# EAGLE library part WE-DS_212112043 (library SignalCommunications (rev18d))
WE-DS D-SUB-Filter Connectors Bent 90° Characteristics Standard type filtered with 1000 pF High attenuation of more than 40 dB @ 180 MHz Choice of earthing metal sheet or high speed earthing clip Rated voltage: 100 VDC Rated current @ 20 ºC: 5 A Withstand voltage: 250 VRMS Insulation resistance: min. 1000 MΩ Operating temperature: –55 ºC to +125 ºC Applications Filtering of interfaces External connection to -printer -sensor -display Details see: http://katalog.we-online.de/en/pbs/Filter_abgewinkelt Created on 2015-05-04 2015 (C) Wurth Elektronik
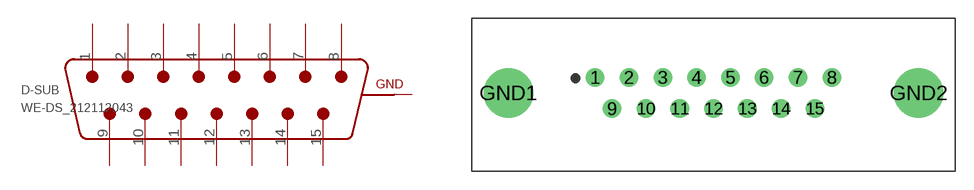
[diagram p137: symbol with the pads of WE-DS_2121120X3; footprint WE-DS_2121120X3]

Designator prefix D-SUB

## WE-DS_212112043 (WE-NUMBER: 212112043/15pins_male)  [WE-DS_2121120X3]
1  1  pas
2  2  pas
3  3  pas
4  4  pas
5  5  pas
6  6  pas
7  7  pas
8  8  pas
9  9  pas
10  10  pas
11  11  pas
12  12  pas
13  13  pas
14  14  pas
15  15  pas
GND1  GND  pas
GND2  GND  pas

## Footprint WE-DS_2121120X3 (pad centres in mm)
drill 1: 1 -9.6,1.27; 2 -6.86,1.27; 3 -4.11,1.27; 4 -1.37,1.27; 5 1.37,1.27; 6 4.11,1.27; 7 6.86,1.27; 8 9.6,1.27; 9 -8.23,-1.27; 10 -5.48,-1.27; 11 -2.74,-1.27; 12 0,-1.27; 13 2.74,-1.27; 14 5.48,-1.27; 15 8.23,-1.27
drill 3: GND1 -16.65,0; GND2 16.65,0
